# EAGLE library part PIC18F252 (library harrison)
PIC18F252 microcontroller
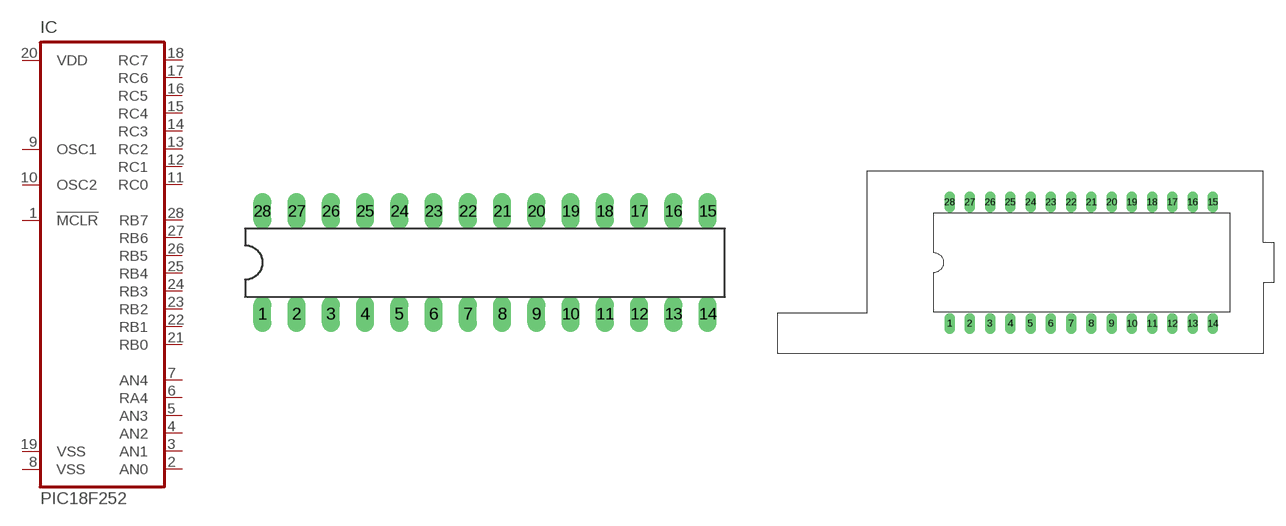
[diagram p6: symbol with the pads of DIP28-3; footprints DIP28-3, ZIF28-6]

Designator prefix IC

## PIC18F252  [DIP28-3]
1  !MCLR  in
2  AN0
3  AN1
4  AN2
5  AN3
6  RA4
7  AN4
8  VSS  pwr
9  OSC1
10  OSC2
11  RC0
12  RC1
13  RC2
14  RC3
15  RC4
16  RC5
17  RC6
18  RC7
19  VSS  pwr
20  VDD  pwr
21  RB0
22  RB1
23  RB2
24  RB3
25  RB4
26  RB5
27  RB6
28  RB7

## PIC18F252ZIF  [ZIF28-6]
Pads as for DIP28-3

## Footprint DIP28-3 (pad centres in mm)
drill 0.813 long: 1 -16.51,-3.81; 2 -13.97,-3.81; 3 -11.43,-3.81; 4 -8.89,-3.81; 5 -6.35,-3.81; 6 -3.81,-3.81; 7 -1.27,-3.81; 8 1.27,-3.81; 9 3.81,-3.81; 10 6.35,-3.81; 11 8.89,-3.81; 12 11.43,-3.81; 13 13.97,-3.81; 14 16.51,-3.81; 15 16.51,3.81; 16 13.97,3.81; 17 11.43,3.81; 18 8.89,3.81; 19 6.35,3.81; 20 3.81,3.81; 21 1.27,3.81; 22 -1.27,3.81; 23 -3.81,3.81; 24 -6.35,3.81; 25 -8.89,3.81; 26 -11.43,3.81; 27 -13.97,3.81; 28 -16.51,3.81

## Footprint ZIF28-6 (pad centres in mm)
drill 0.813 long: 1 -16.51,-7.62; 2 -13.97,-7.62; 3 -11.43,-7.62; 4 -8.89,-7.62; 5 -6.35,-7.62; 6 -3.81,-7.62; 7 -1.27,-7.62; 8 1.27,-7.62; 9 3.81,-7.62; 10 6.35,-7.62; 11 8.89,-7.62; 12 11.43,-7.62; 13 13.97,-7.62; 14 16.51,-7.62; 15 16.51,7.62; 16 13.97,7.62; 17 11.43,7.62; 18 8.89,7.62; 19 6.35,7.62; 20 3.81,7.62; 21 1.27,7.62; 22 -1.27,7.62; 23 -3.81,7.62; 24 -6.35,7.62; 25 -8.89,7.62; 26 -11.43,7.62; 27 -13.97,7.62; 28 -16.51,7.62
